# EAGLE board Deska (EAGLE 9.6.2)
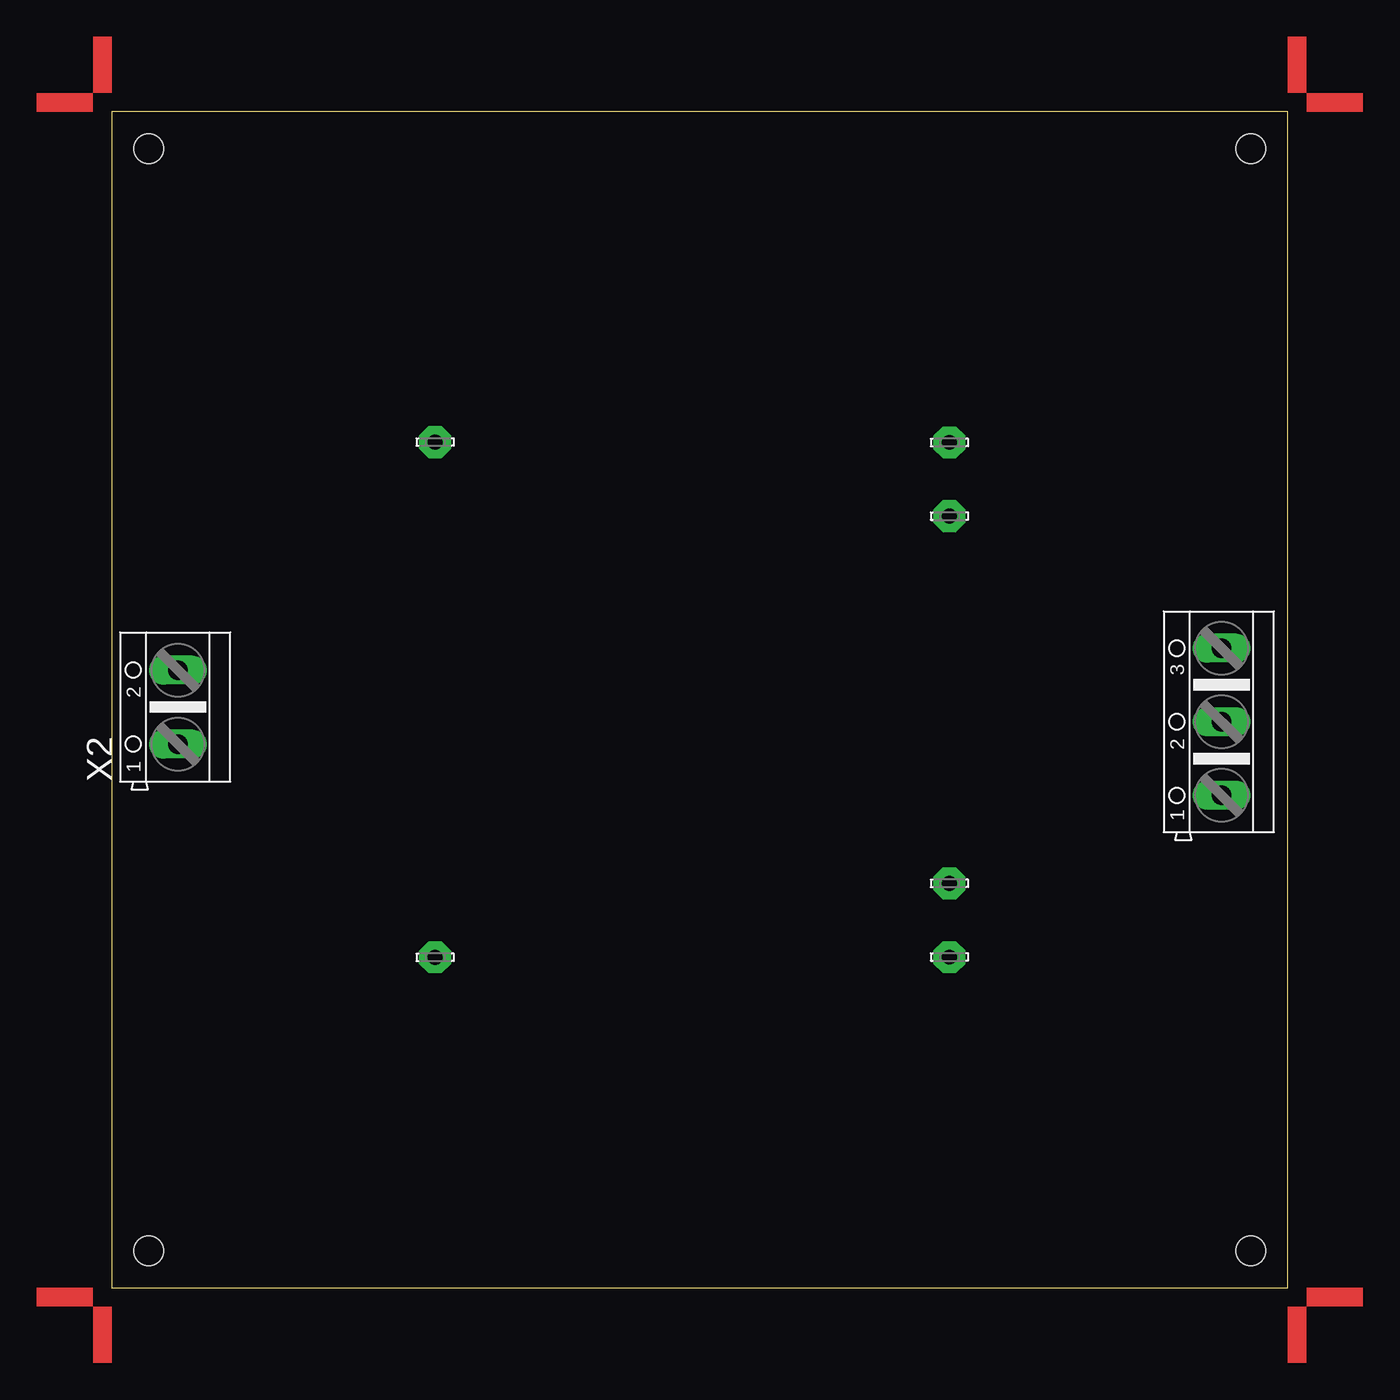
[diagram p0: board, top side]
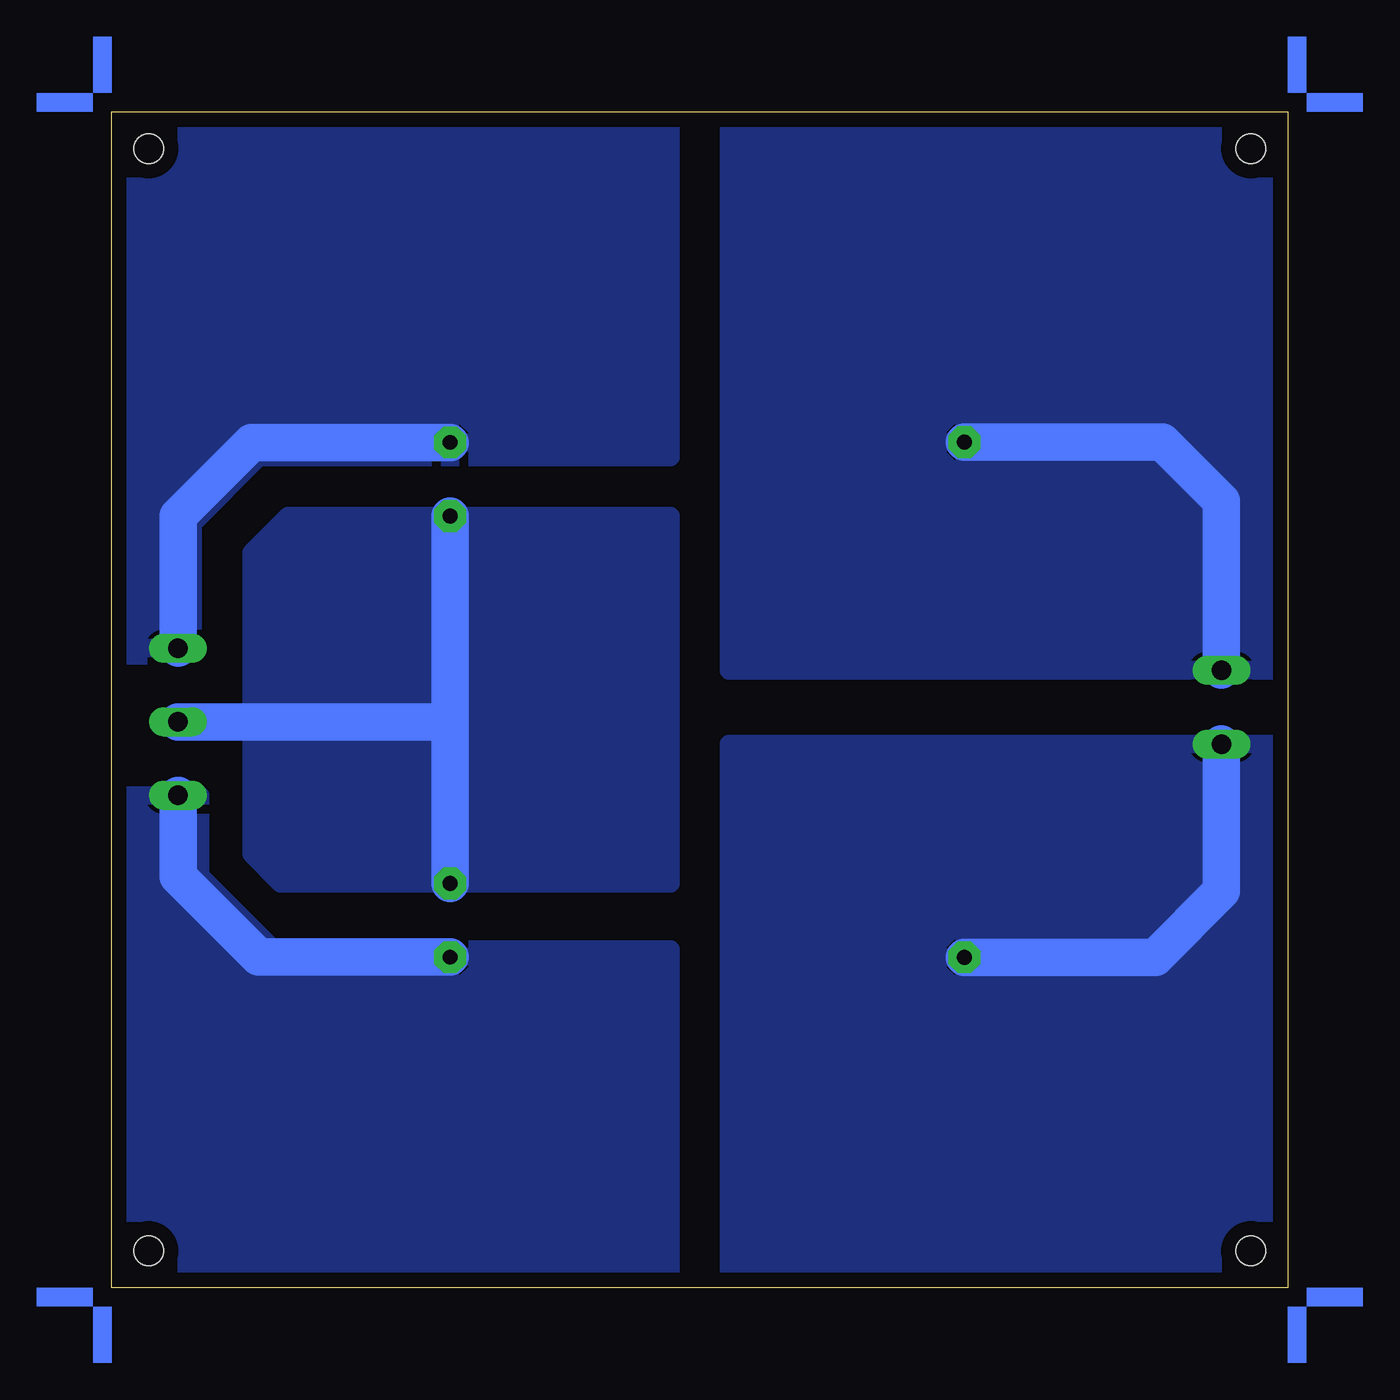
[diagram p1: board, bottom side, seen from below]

Size 80 x 80 mm. Coordinates in mm from the lower left corner, seen from the top.
Outline: 0,0 80,0 80,80 0,80 0,0
Copper layers (1*16): Top 0.035mm / dielectric 1.5mm / Bottom 0.035mm
Design rules "default": minimum track width 6mil, minimum drill 0.35mm, track to track 6mil, track to pad 6mil, pad to pad 6mil, via to via 6mil, smd to smd 6mil, copper to edge 40mil, drill to drill 6mil, minimum pad ring 10mil, minimum via ring 8mil, stop-mask expansion 4mil, vias tented up to drill 0mil, thermal gap 10mil
Holes 2 mm at 2.5,77.5 77.5,77.5 77.5,2.5 2.5,2.5

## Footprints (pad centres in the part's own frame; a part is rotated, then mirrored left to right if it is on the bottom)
LSP10 = drill 1.016 pad 2.159 octagon: MP 0,0
AK500/3 = drill 1.321 long: 1 -5.004,0; 2 0,0; 3 5.004,0
AK500/2 = drill 1.321 long: 1 -2.515,0; 2 2.515,0

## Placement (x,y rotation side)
LSP1  LSP10  [LSP10]  21.99,22.48 0 top
LSP2  LSP10  [LSP10]  21.99,57.53 0 top
LSP3  LSP10  [LSP10]  56.99,57.51 0 top
LSP4  LSP10  [LSP10]  56.99,27.51 0 top
LSP5  LSP10  [LSP10]  56.99,52.49 0 top
LSP6  LSP10  [LSP10]  56.99,22.49 0 top
U$1  [ANGLE-SW1-16]  80,80 0 top
U$2  [ANGLE-SW1-16]  0,80 90 top
U$3  [ANGLE-SW1-16]  0,0 180 top
U$4  [ANGLE-SW1-16]  80,0 270 top
X1  [AK500/3]  75.5,38.5 90 top
X2  [AK500/2]  4.5,39.5 90 top

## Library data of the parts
LSP1-LSP6 = solpad
U$1-U$4 = marks
X1 X2 = con-ptr500; OC_FARNELL: unknown; OC_NEWARK: unknown

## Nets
N$1: LSP4.MP LSP5.MP X1.2
N$2: LSP3.MP X1.3
N$3: LSP6.MP X1.1
N$4: LSP1.MP X2.1
N$5: LSP2.MP X2.2

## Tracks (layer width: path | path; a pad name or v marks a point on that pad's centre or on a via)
N$1
  Bottom 2.54: LSP5.MP 56.99,38.5 | 56.99,38.5 LSP4.MP | X1.2 56.99,38.5
  pour Bottom (isolate 0.813): 42,52.5 68,52.5 70.5,50 70.5,29.5 68.5,27.5 42,27.5
N$2
  Bottom 2.54: LSP3.MP 70.49,57.51 75.5,52.5 X1.3
  pour Bottom (isolate 0.813): 80,80 80,43 75,43 74.5,43.5 74.5,52 70,56.5 42,56.5 42,80
N$3
  Bottom 2.54: LSP6.MP 69.99,22.49 75.5,28 X1.1
  pour Bottom (isolate 0.813): 80,33.5 74,33.5 74,28 69,23 42,23 42,0 80,0
N$4
  Bottom 2.54: LSP1.MP 9.01,22.48 4.5,26.98 X2.1
  pour Bottom (isolate 0.813): 0,37 38,37 38,0 0,0
N$5
  Bottom 2.54: LSP2.MP 8.52,57.53 4.5,53.52 X2.2
  pour Bottom (isolate 0.813): 0,42 38,42 38,80 0,80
